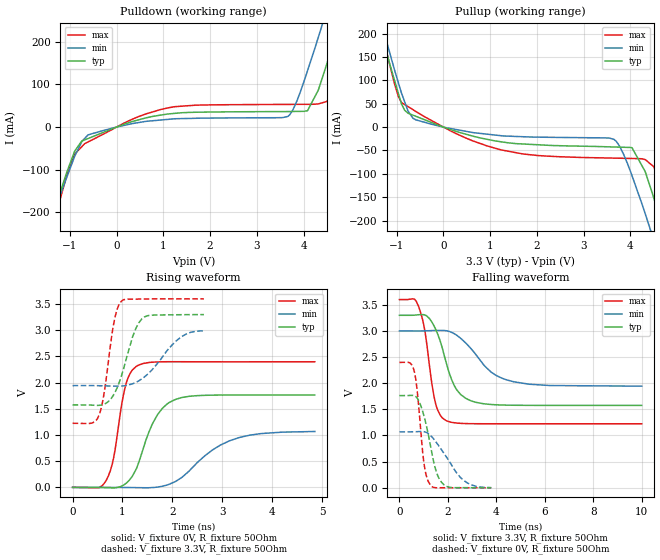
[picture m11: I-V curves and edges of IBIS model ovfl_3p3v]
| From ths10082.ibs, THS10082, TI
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|   ovfl_3p3v Model
[Model]   ovfl_3p3v
Model_type   Output
Polarity   Non-Inverting
Vmeas = 1.65
Vref =  1.65
Cref =  2pF
Rref =  50
|   typ   min   max
C_comp   1.935e-12   1.914e-12   1.989e-12
[Voltage Range]   3.3   3   3.6
|Ambient Temperature   25   85   -40
|Junction Temperature
[Temperature Range]   27   125   -40
[Pullup Reference]   3.3   3   3.6
[Pulldown Reference]   0   0   0
[Power Clamp Reference]   3.3   3   3.6
[GND Clamp Reference]   0   0   0
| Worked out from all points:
|   slope of the pulldown table from 0 to 0.495 V, typ, clamps not added: 28 ohm
|   slope of the pullup table from 0 to 0.495 V, typ, clamps not added: 31.6 ohm
|   falling waveform, V_fixture 3.3V, R_fixture 50Ohm: 20-80 % time 738ps typ, 1.28ns min, 451ps max; typ from 3.3 V to 1.58 V
|   rising waveform, V_fixture 0V, R_fixture 50Ohm: 20-80 % time 444ps typ, 847ps min, 252ps max; typ from 0 V to 1.76 V
|   rising waveform, V_fixture 3.3V, R_fixture 50Ohm: 20-80 % time 334ps typ, 567ps min, 210ps max; typ from 1.58 V to 3.3 V
|   falling waveform, V_fixture 0V, R_fixture 50Ohm: 20-80 % time 503ps typ, 942ps min, 293ps max; typ from 1.76 V to 0 V
[Pulldown]
|   Voltage   I(typ)   I(min)   I(max)
-3.3V     -968.4mA   -894.2mA   -1.061A
-1.429V   -233.2mA   -231.1mA   -258.1mA
-897.6mV  -56.98mA   -69.25mA   -63.82mA
-591mV    -26.14mA   -17.74mA   -33.87mA
1.091V    30.64mA    17.97mA    44.81mA
3.663V    36.44mA    24.94mA    53.22mA
4.085V    38.35mA    132.1mA    53.44mA
4.316V    86.63mA    210.5mA    54.32mA
4.468V    137.7mA    264.4mA    59.09mA
4.68V     216.9mA    341.1mA    106.3mA
5.119V    383.4mA    505mA      272.9mA
6.6V      977.1mA    1.079A     886.7mA
[Pullup]
|   Voltage   I(typ)   I(min)   I(max)
-3.3V     1.016A     996.7mA    1.053A
-1.386V   226.3mA    245.9mA    228.4mA
-961.2mV  71.32mA    94.07mA    65.04mA
-828.3mV  35.84mA    53.8mA     48.18mA
-591mV    23.07mA    15.52mA    33.53mA
1.246V    -31.72mA   -18.61mA   -49.05mA
3.645V    -42.63mA   -26.18mA   -66.44mA
4.036V    -44.49mA   -104.4mA   -67.21mA
4.468V    -141.3mA   -232.1mA   -82.15mA
4.709V    -223.2mA   -311.8mA   -144.6mA
4.867V    -277.7mA   -364.9mA   -205mA
6.6V      -951.9mA   -980.9mA   -925.5mA
[Ramp]
R_load = 50
|   typ   min   max
dV/dt_r   1.05825/4.41742e-10   0.642047/8.42672e-10   1.43893/2.50443e-10
dV/dt_f   1.0345/7.3735e-10   0.633808/1.27442e-09   1.42541/4.50335e-10
[Falling Waveform]
V_fixture = 3.3V
V_fixture_min = 3V
V_fixture_max = 3.6V
R_fixture = 50Ohm
|   Time   V(typ)   V(min)   V(max)
0s        3.3V       3V         3.6V
788ps     3.31V      3V         3.474V
1.056ns   3.305V     3.002V     2.987V
1.482ns   3.044V     3.009V     1.633V
1.936ns   2.385V     3.004V     1.283V
2.38ns    1.866V     2.912V     1.237V
3.19ns    1.631V     2.527V     1.225V
3.776ns   1.593V     2.216V     1.225V
4.726ns   1.579V     2.027V     1.224V
9.998ns   1.576V     1.944V     1.224V
[Rising Waveform]
V_fixture = 0V
V_fixture_min = 0V
V_fixture_max = 0V
R_fixture = 50Ohm
|   Time   V(typ)   V(min)   V(max)
0s        1.442nV    2.279nV    1.234nV
518ps     -1.207mV   197.8uV    -7.146mV
678ps     -5.5mV     232.4uV    141mV
824ps     -8.845mV   -94uV      568.6mV
1.078ns   81.48mV    -2.198mV   1.999V
1.288ns   377.4mV    -5.016mV   2.318V
1.696ns   1.379V     4.277mV    2.396V
2.068ns   1.681V     115.4mV    2.4V
3.148ns   1.764V     890.7mV    2.398V
4.854ns   1.764V     1.067V     2.398V
[Rising Waveform]
V_fixture = 3.3V
V_fixture_min = 3V
V_fixture_max = 3.6V
R_fixture = 50Ohm
|   Time   V(typ)   V(min)   V(max)
0s        1.576V     1.943V     1.224V
386ps     1.571V     1.943V     1.227V
534ps     1.567V     1.941V     1.385V
634ps     1.589V     1.939V     1.809V
842ps     1.799V     1.933V     3.212V
978ps     2.125V     1.936V     3.555V
1.246ns   2.984V     1.995V     3.595V
1.418ns   3.243V     2.092V     3.597V
2.098ns   3.297V     2.815V     3.6V
2.632ns   3.3V       2.991V     3.6V
[Falling Waveform]
V_fixture = 0V
V_fixture_min = 0V
V_fixture_max = 0V
R_fixture = 50Ohm
|   Time   V(typ)   V(min)   V(max)
0s        1.764V     1.07V      2.398V
428ps     1.766V     1.07V      2.391V
608ps     1.763V     1.071V     2.236V
736ps     1.714V     1.073V     1.843V
998ps     1.398V     1.074V     522mV
1.27ns    832.9mV    1.008V     56.74mV
1.526ns   301.2mV    865.4mV    -833.9uV
1.82ns    64.37mV    671.9mV    693.2uV
2.638ns   1.837mV    145.8mV    182uV
3.788ns   237.7uV    2.905mV    130.7uV
